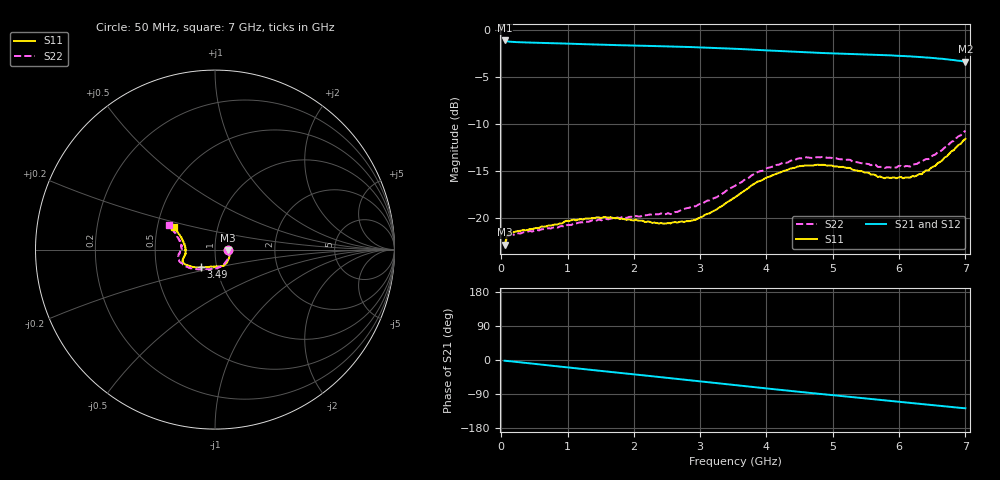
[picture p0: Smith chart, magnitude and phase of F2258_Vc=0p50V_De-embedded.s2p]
! Integrated Device Technology
! Corporate Headquarters
! 6024 Silver Creek Valley Road
! San Jose, CA 95138  USA
! Phone:  1-408-284-8200
! Toll Free:  1-800-223-1366
! Webpage:  http://www.idt.com/
! Timing and RF Division
! 515 Groton Road, Suite 102
! Westford, MA 01886-6024
! Device:  F2258
! Description: Voltage Variable RF Attenuator
! Frequency:  50.0 -  6000.00 MHz
! Package:  3x3 mm Thin QFN Plastic Package: 16 pin
! Ports:  2 RF, 2 DC
!  Pin  1  = NC
!  Pin  2  = NC
!  Pin  3  = RF2  = Port 2
!  Pin  4  = GND
!  Pin  5  = Vdd
!  Pin  6  = NC
!  Pin  7  = VCTRL
!  Pin  8  = NC
!  Pin  9  = GND
!  Pin 10  = RF1  = Port 1
!  Pin 11  = NC
!  Pin 12  = NC
!  Pin 13  = NC
!  Pin 14  = NC
!  Pin 15  = NC
!  Pin 16  = NC
! Vcntrl:  0.500 Volts
! Vdd:  +3.300 Volts
! Current:  1.096 mA
! Data:  The device was measured on a the F2258 evaluation board which has
!  individual transmission lines to the RF pins.  Data was collected
!  using a calibrated network analyzer.  The evaluation board was
!  de-embedded using a TRL calibration technique.
!  The reference plane is the edge of the package pin.
! Misc:  SN 10
!  Action Tracker AT0285
! Date Measured:  2014-12-10
! Date:  2016-01-13  MJV
! Note:
!  Integrated Device Technology supplies this data as a sample of measured
!  data at the package pin for this product.  Your particular data for this
!  product may vary.
!  Data was taken at 25 degrees C.
!  Integrated Device Technology reserves the right to change this data at anytime.
!Freq_(GHz)  S11M_(dB)  S11P_(deg)  S21M_(dB)  S21P_(deg)  S12M_(dB)  S12P_(deg)  S22M_(dB)  S22P_(deg)
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# GHz S dB R 50
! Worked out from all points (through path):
!   201 points, 50 MHz to 7 GHz, reference 50 ohm
!   highest |S21| = -1.10 dB at 50 MHz (marker M1); lowest = -3.4 dB at 7 GHz (marker M2)
!   group delay of S21, straight-line fit = 50.5 ps
!   lowest |S11| = -22.8 dB at 50 MHz (marker M3), VSWR 1.16, Z = 57.8 - j0.448 ohm
!   |S11| at or under -10 dB: start of sweep to end of sweep
!   |S22| runs from -23.0 to -10.7 dB; largest |S21 - S12| = 0.00059
!   S11 on the Smith chart (normalised r, x): 50 MHz: 1.16, -0.01; 3.49 GHz: 0.84, -0.17; 7 GHz: 0.61, +0.17
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0.05  -22.83 -3.1  -1.10 -2.0  -1.10 -2.0  -22.97 -3.1
0.08475  -21.92 -5.0  -1.19 -2.5  -1.19 -2.5  -22.09 -5.0
0.15425  -21.48 -7.8  -1.25 -3.7  -1.25 -3.7  -21.73 -8.6
0.71025  -20.78 -31.9  -1.39 -14.1  -1.38 -14.1  -21.06 -35.4
1.2315  -20.13 -52.2  -1.49 -23.8  -1.49 -23.8  -20.43 -59.2
1.6485  -19.89 -63.2  -1.58 -31.5  -1.58 -31.4  -20.04 -72.2
2.37825  -20.55 -82.7  -1.71 -44.8  -1.71 -44.8  -19.57 -90.7
2.552  -20.55 -88.4  -1.74 -48.0  -1.74 -48.0  -19.57 -96.0
2.93425  -20.15 -104.9  -1.82 -55.1  -1.82 -55.1  -18.73 -109.6
3.247  -19.07 -118.5  -1.90 -61.0  -1.90 -61.0  -17.78 -122.0
3.49025  -17.93 -129.1  -1.97 -65.6  -1.97 -65.6  -16.69 -131.3
3.525  -17.78 -130.2  -1.98 -66.2  -1.98 -66.2  -16.56 -132.8
4.0115  -15.65 -145.6  -2.16 -75.3  -2.17 -75.3  -14.66 -148.8
4.46325  -14.52 -154.7  -2.32 -83.4  -2.33 -83.4  -13.68 -160.2
4.7065  -14.39 -158.1  -2.39 -87.7  -2.40 -87.7  -13.58 -164.6
5.2625  -14.66 -164.7  -2.55 -97.4  -2.55 -97.4  -13.80 -172.9
5.6795  -15.62 -171.0  -2.63 -104.6  -2.64 -104.6  -14.55 -178.5
5.85325  -15.71 -175.2  -2.69 -107.8  -2.69 -107.8  -14.59 176.8
6.166  -15.69 176.8  -2.79 -113.3  -2.80 -113.3  -14.52 170.7
6.33975  -15.33 170.0  -2.87 -116.4  -2.88 -116.4  -14.02 166.2
6.722  -13.42 157.1  -3.11 -123.1  -3.11 -123.1  -12.41 157.0
7  -11.56 150.9  -3.35 -127.4  -3.36 -127.4  -10.69 152.0
